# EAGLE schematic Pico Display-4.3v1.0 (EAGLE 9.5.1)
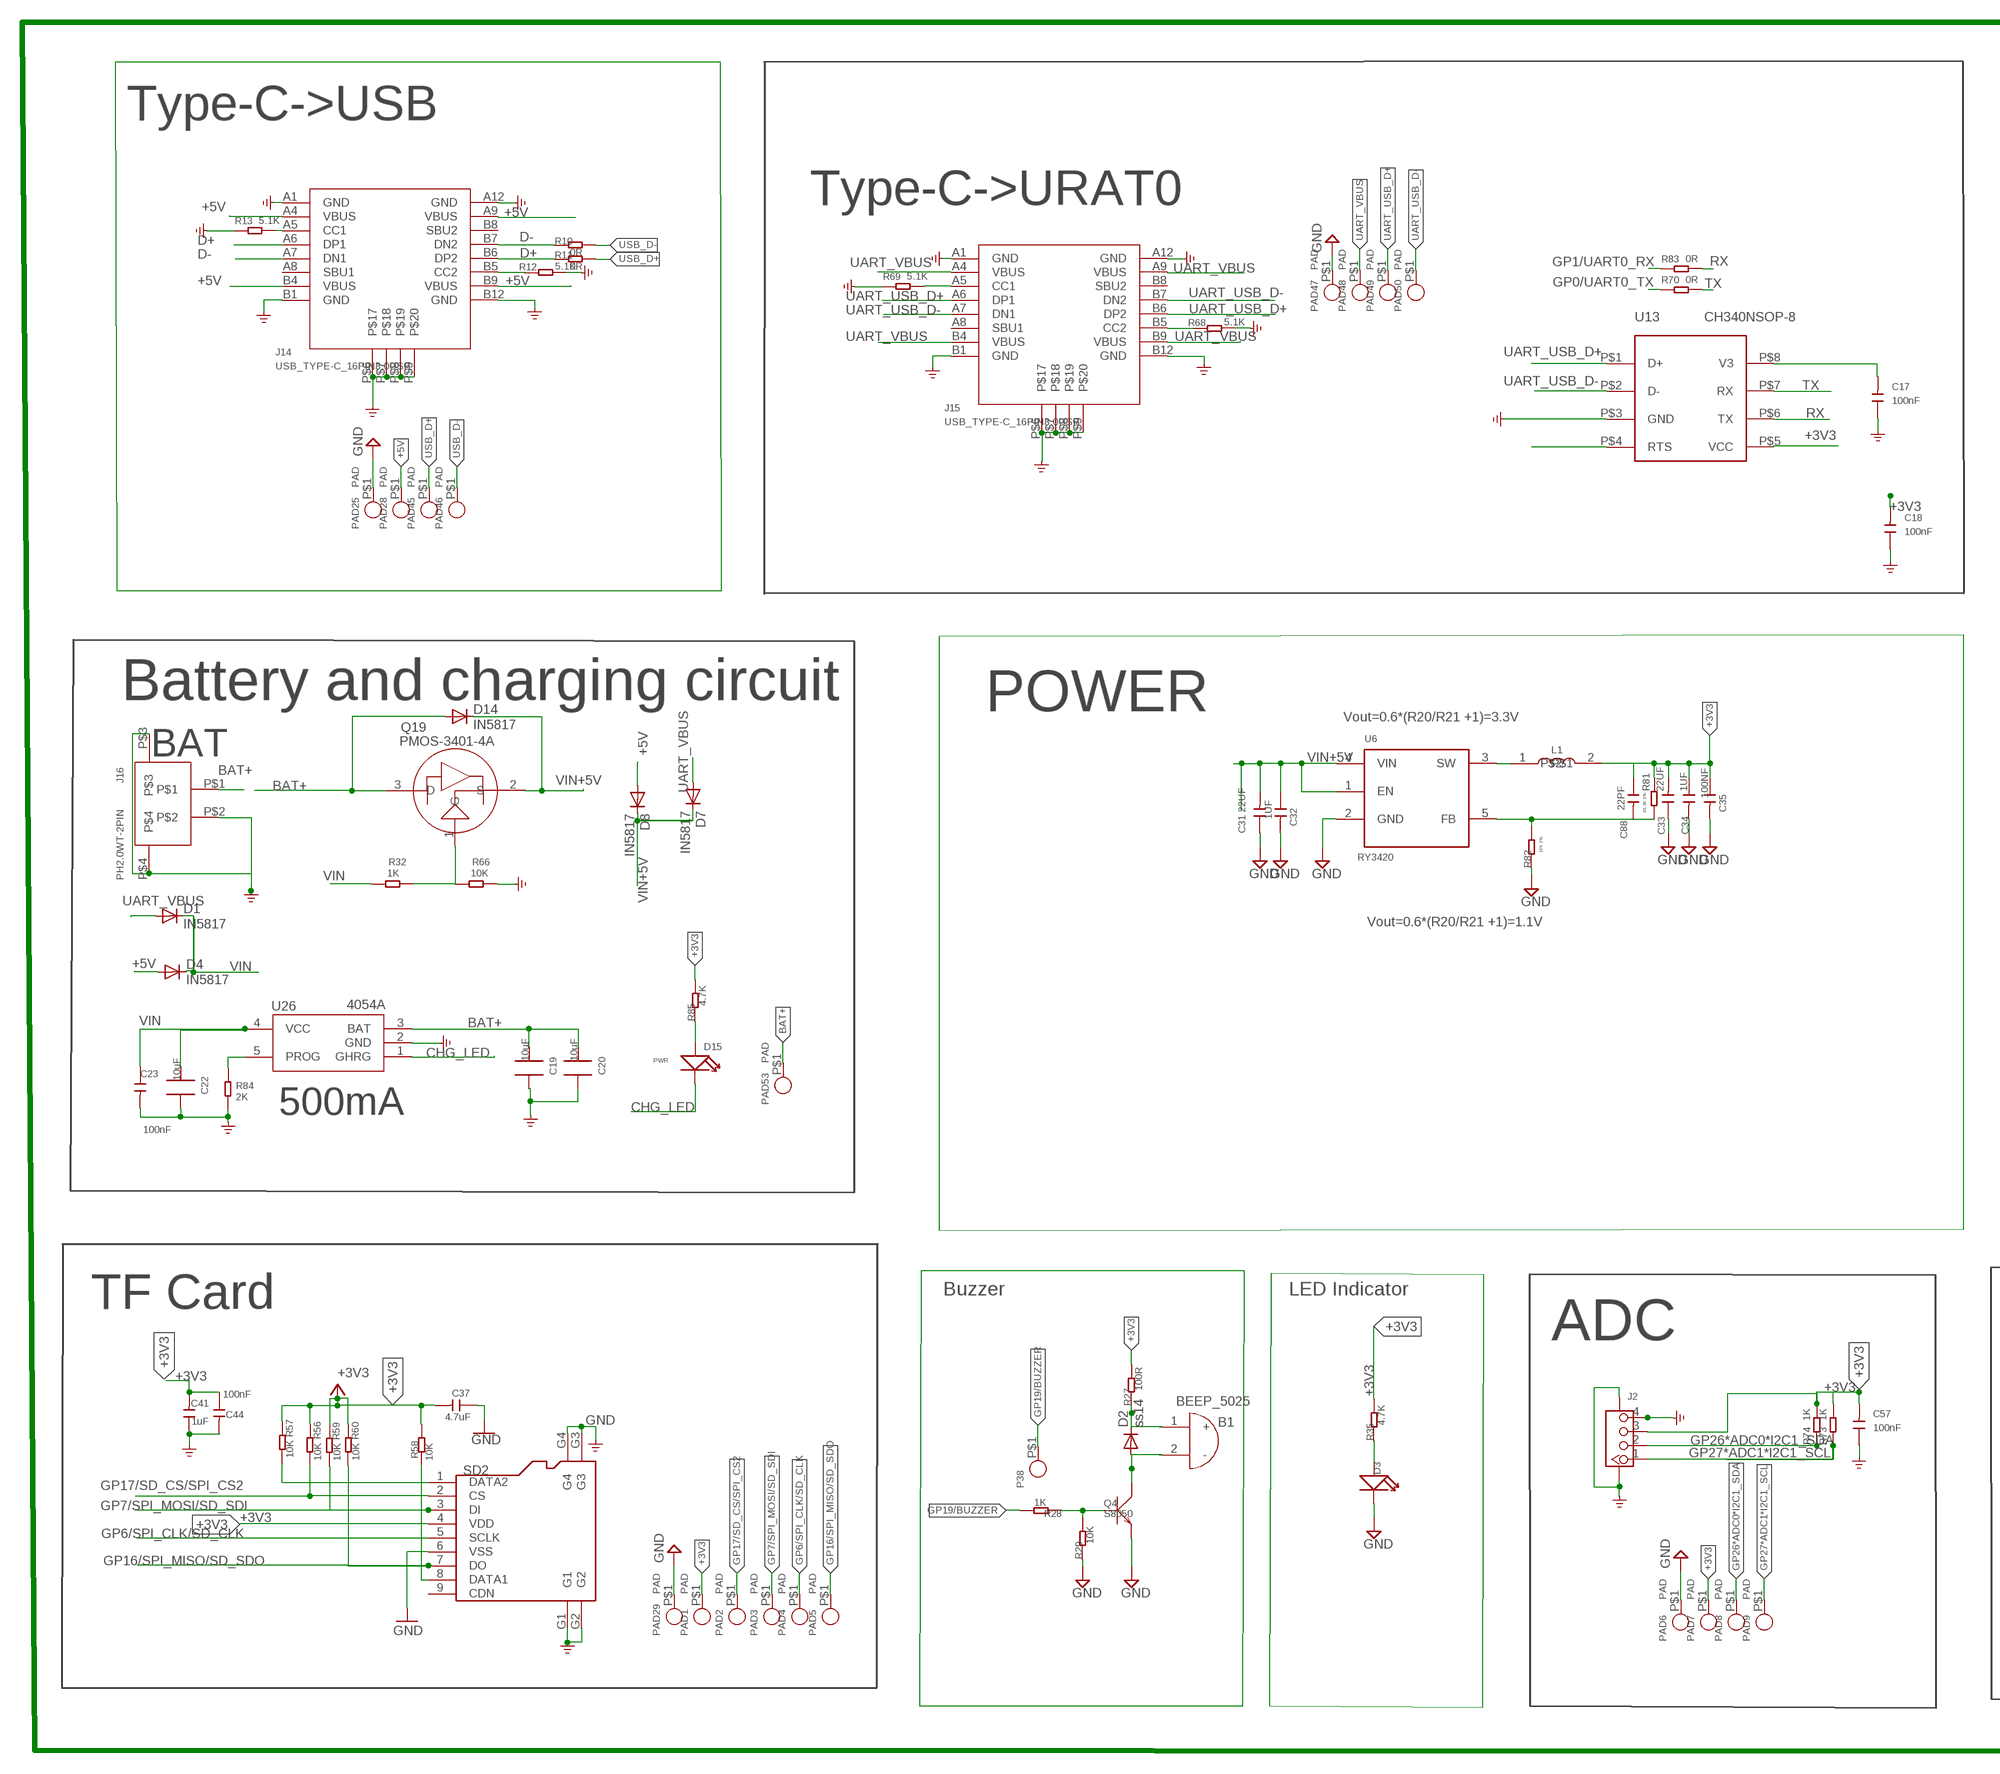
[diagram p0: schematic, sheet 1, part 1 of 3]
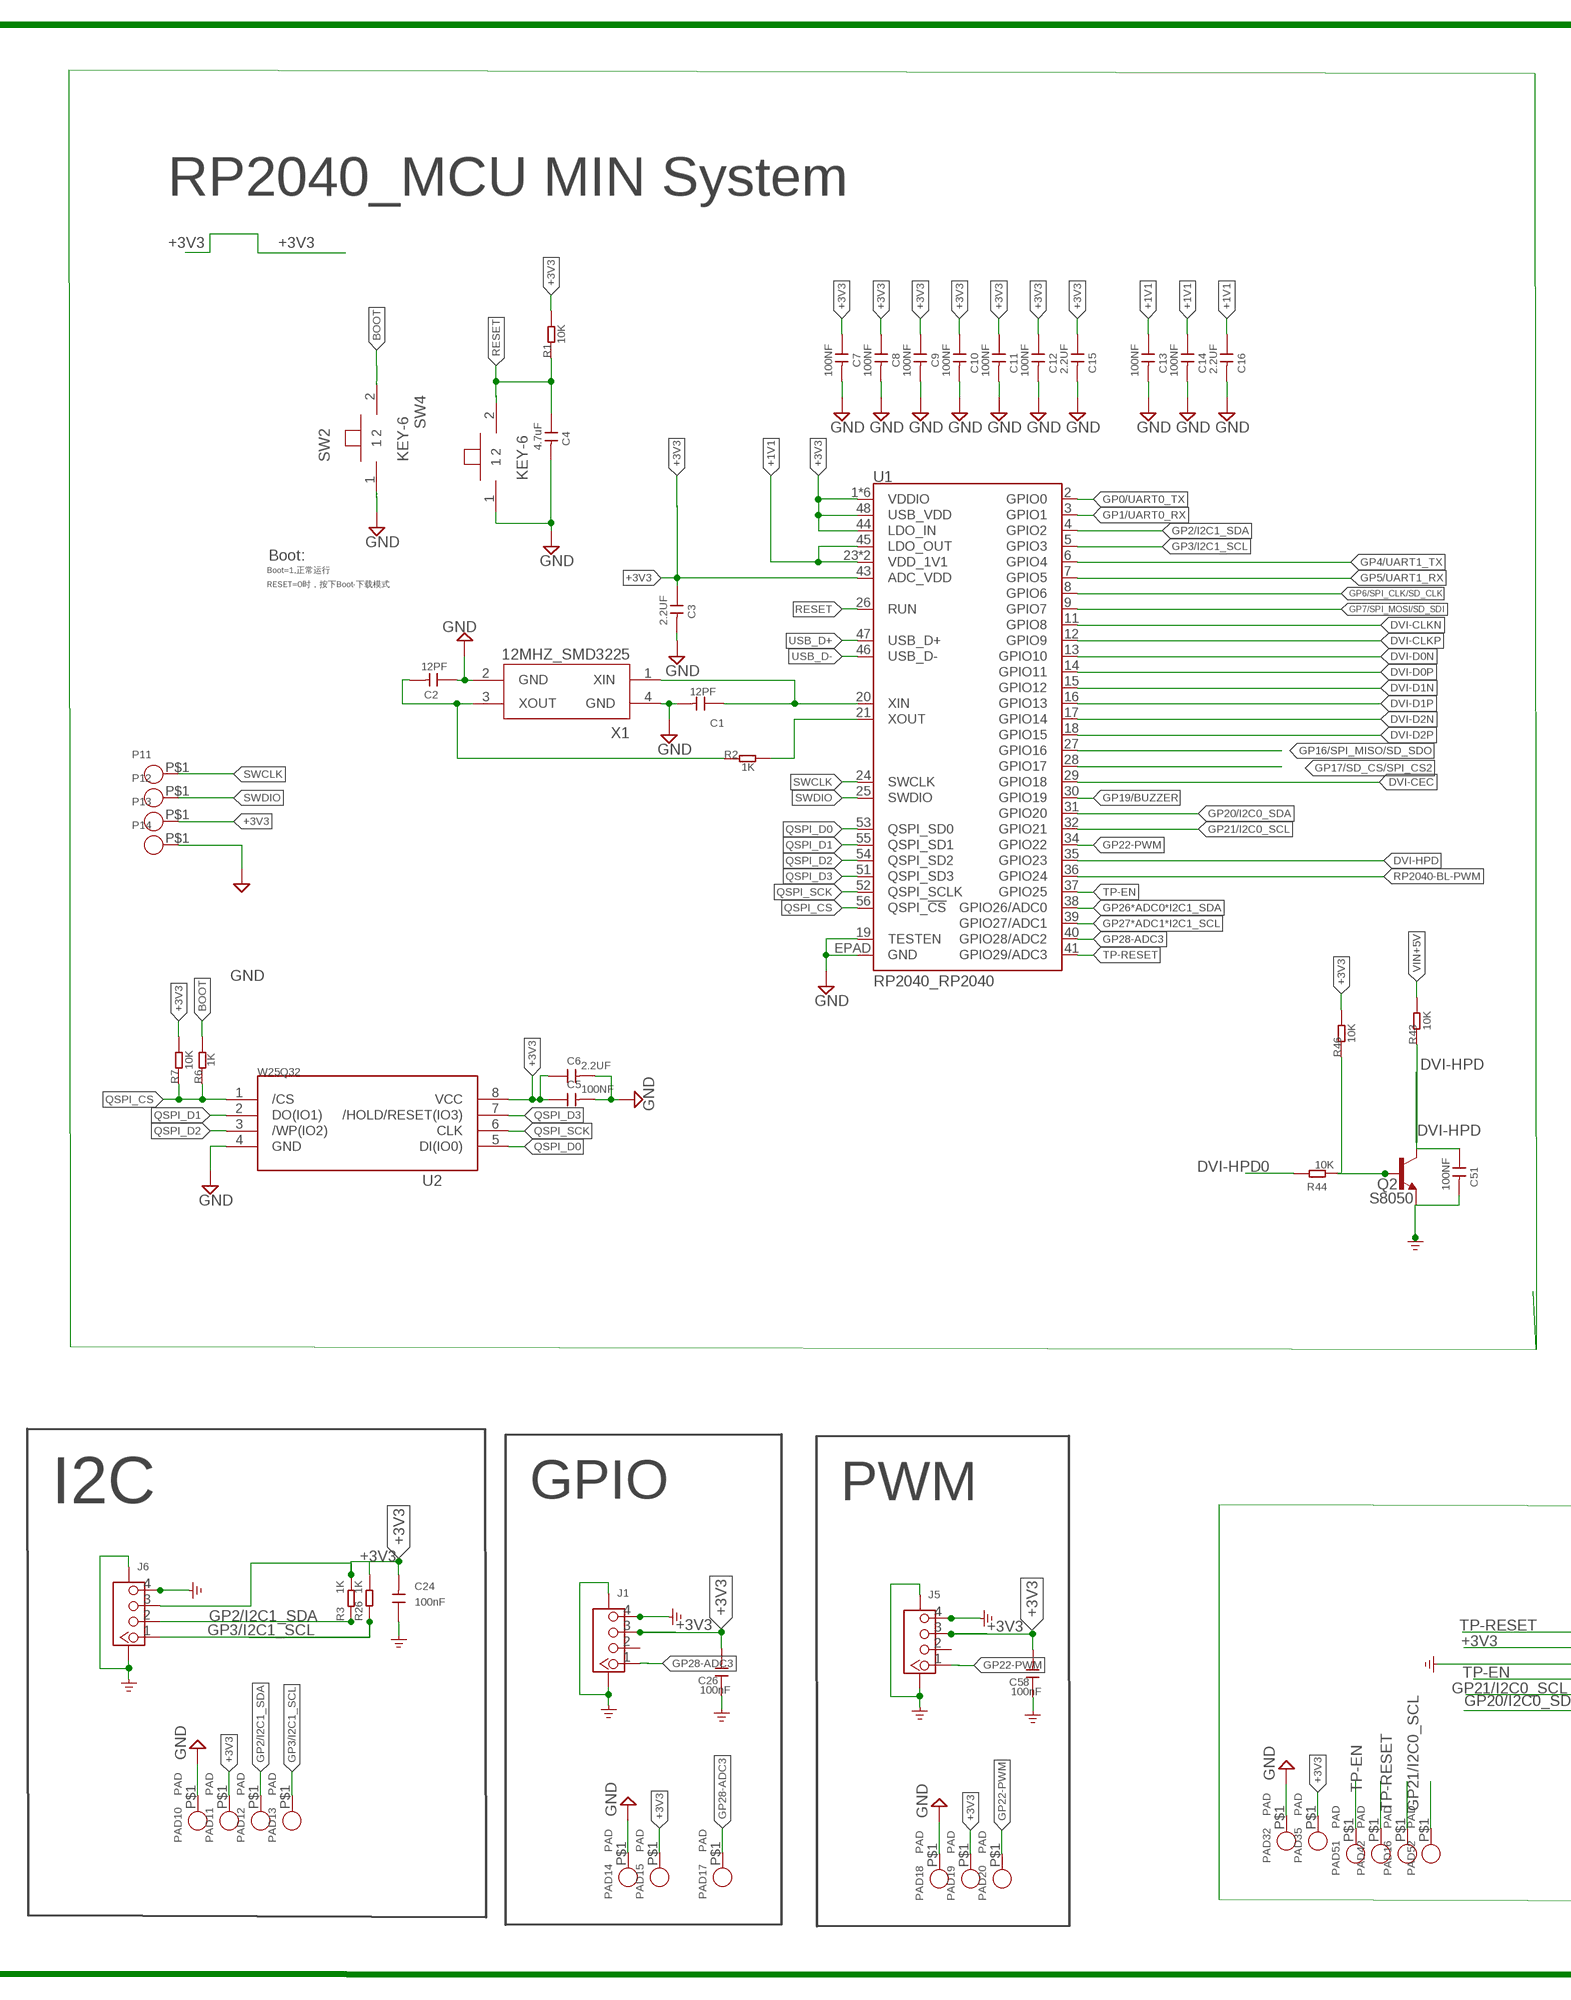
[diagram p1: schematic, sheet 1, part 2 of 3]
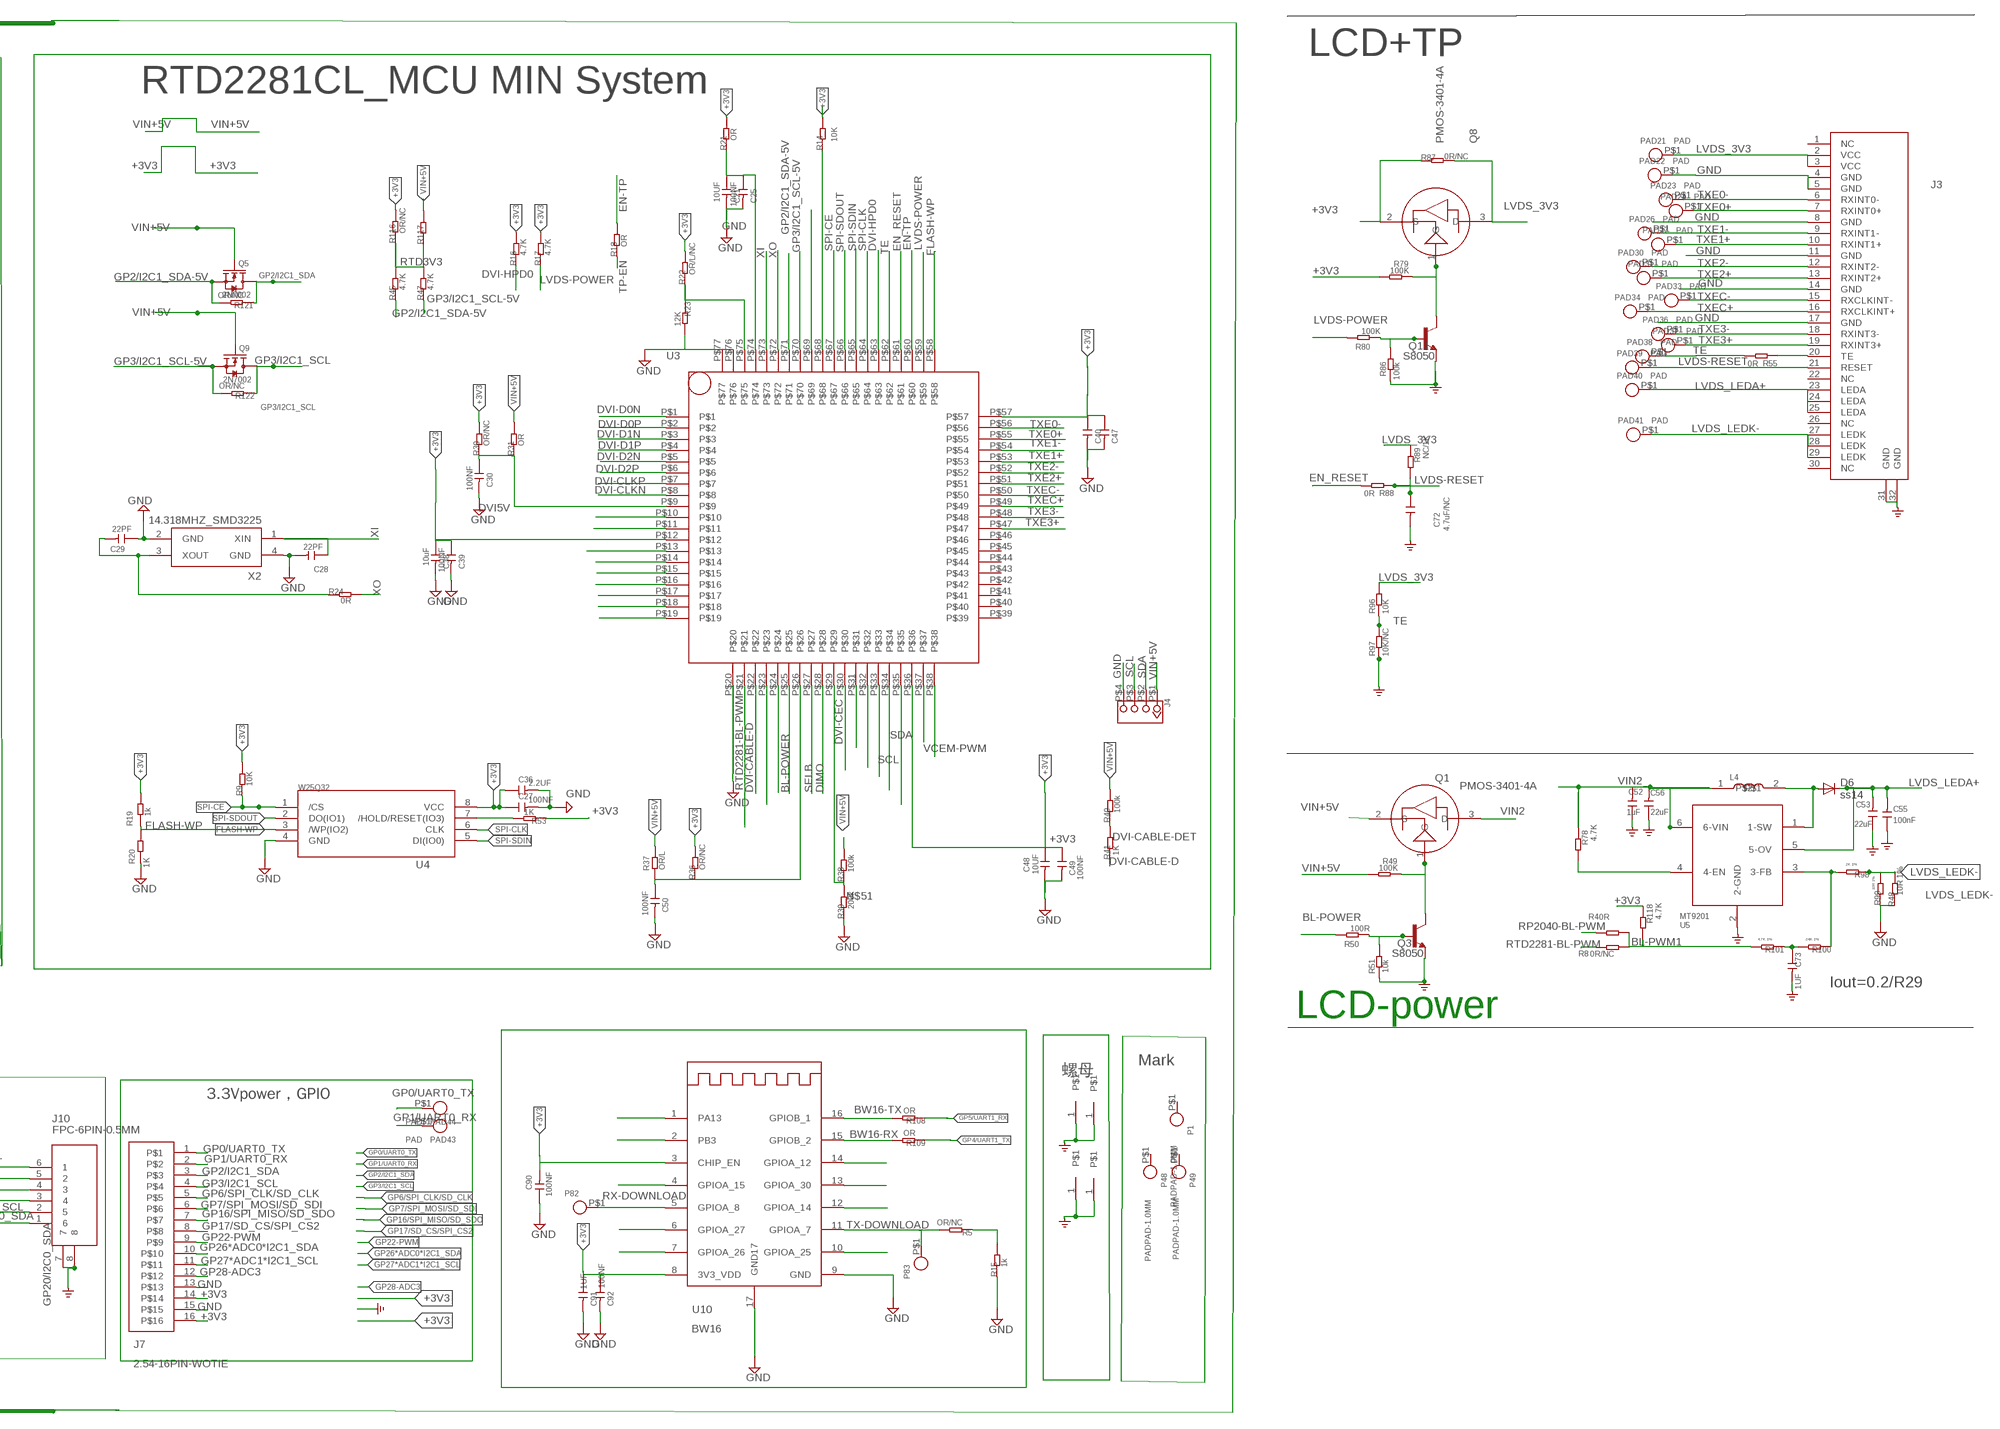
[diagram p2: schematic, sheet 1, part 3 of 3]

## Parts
B1  BEEP_5025  [BEEP_5025]
C1  12PF  A_XBJ_C0603  [A_XBJ_0603]
C2  12PF  A_XBJ_C0603  [A_XBJ_0603]
C3  2.2UF  A_XBJ_C0603  [A_XBJ_0603]
C4  4.7uF  A_XBJ_C0603  [A_XBJ_0603]
C5  100NF  A_XBJ_C0603  [A_XBJ_0603]
C6  2.2UF  A_XBJ_C0603  [A_XBJ_0603]
C7  100NF  A_XBJ_C0603  [A_XBJ_0603]
C8  100NF  A_XBJ_C0603  [A_XBJ_0603]
C9  100NF  A_XBJ_C0603  [A_XBJ_0603]
C10  100NF  A_XBJ_C0603  [A_XBJ_0603]
C11  100NF  A_XBJ_C0603  [A_XBJ_0603]
C12  100NF  A_XBJ_C0603  [A_XBJ_0603]
C13  100NF  A_XBJ_C0603  [A_XBJ_0603]
C14  100NF  A_XBJ_C0603  [A_XBJ_0603]
C15  2.2UF  A_XBJ_C0603  [A_XBJ_0603]
C16  2.2UF  A_XBJ_C0603  [A_XBJ_0603]
C17  100nF  C0603  [0603]
C18  100nF  C0603  [0603]
C19  10uF  C0805_S  [0805_S]
C20  10uF  C0805_S  [0805_S]
C21  10UF  A_XBJ_C0603  [A_XBJ_0603]
C22  10uF  C0805_S  [0805_S]
C23  100nF  C-0603  [C0603]
C24  100nF  C0603  [0603]
C25  100NF  A_XBJ_C0603  [A_XBJ_0603]
C26  100nF  C0603  [0603]
C27  100NF  A_XBJ_C0603  [A_XBJ_0603]
C28  22PF  A_XBJ_C0603  [A_XBJ_0603]
C29  22PF  A_XBJ_C0603  [A_XBJ_0603]
C30  100NF  A_XBJ_C0603  [A_XBJ_0603]
C31  22UF  A_XBJ_C0805  [A_XBJ_0805]
C32  1UF  A_XBJ_C0603  [A_XBJ_0603]
C33  22UF  A_XBJ_C0805  [A_XBJ_0805]
C34  1UF  A_XBJ_C0603  [A_XBJ_0603]
C35  100NF  A_XBJ_C0603  [A_XBJ_0603]
C36  2.2UF  A_XBJ_C0603  [A_XBJ_0603]
C37  4.7uF  DISCRETE_C-0603  [DISCRETE_C0603]
C38  10uF  A_XBJ_C0603  [A_XBJ_0603]
C39  100NF  A_XBJ_C0603  [A_XBJ_0603]
C40  10UF  A_XBJ_C0603  [A_XBJ_0603]
C41  1uF  DISCRETE_C-0603  [DISCRETE_C0603]
C44  100nF  C-0603  [C0603]
C47  100NF  A_XBJ_C0603  [A_XBJ_0603]
C48  10UF  A_XBJ_C0603  [A_XBJ_0603]
C49  100NF  A_XBJ_C0603  [A_XBJ_0603]
C50  100NF  A_XBJ_C0603  [A_XBJ_0603]
C51  100NF  A_XBJ_C0603  [A_XBJ_0603]
C52  1uF  C0603  [0603]
C53  22uF  C0805  [0805]
C55  100nF  C0603  [0603]
C56  22uF  C0805  [0805]
C57  100nF  C0603  [0603]
C58  100nF  C0603  [0603]
C72  4.7uF/NC  C0603  [0603]
C73  1UF  A_XBJ_C0603  [A_XBJ_0603]
C88  22PF  A_XBJ_C0603  [A_XBJ_0603]
C90  100NF  A_XBJ_C0603  [A_XBJ_0603]
C91  1UF  A_XBJ_C0603  [A_XBJ_0603]
C92  100NF  A_XBJ_C0603  [A_XBJ_0603]
D1  IN5817  DIODE-DO-214AC  [DO-214AC]
D2  ss14  DIODE-DO-214AC  [DO-214AC]
D3  DISCRETE_007-LED0603  [DISCRETE_D0603]
D4  IN5817  DIODE-DO-214AC  [DO-214AC]
D6  ss14  DIODE-DO-214AC  [DO-214AC]
D7  IN5817  DIODE-DO-214AC  [DO-214AC]
D8  IN5817  DIODE-DO-214AC  [DO-214AC]
D14  IN5817  DIODE-DO-214AC  [DO-214AC]
D15  DISCRETE_007-LED0603  [DISCRETE_D0603]
J1  CONNECTOR_TWIG-4P-2.0-SMD-FEMALE-REINFORCE90D  [CONNECTOR_4P-SMD-2.0-90D]
J2  CONNECTOR_TWIG-4P-2.0-SMD-FEMALE-REINFORCE90D  [CONNECTOR_4P-SMD-2.0-90D]
J3  FPC-0.5-30P-LVDS  [FPC-30P-0.5]
J4  CON_4PIN_DIP_P2.54  [CON_4PIN_DIP_P2.54]
J5  CONNECTOR_TWIG-4P-2.0-SMD-FEMALE-REINFORCE90D  [CONNECTOR_4P-SMD-2.0-90D]
J6  CONNECTOR_TWIG-4P-2.0-SMD-FEMALE-REINFORCE90D  [CONNECTOR_4P-SMD-2.0-90D]
J7  2.54-16PIN-WOTIE  [2.54-16P-WOTIE]
J10  FPC-6PIN-0.5MM  [FPC-6PIN-0.5MM]
J14  USB_TYPE-C_16PIN3.0USB  [KEVIN_3.0TYPEC-SMD]
J15  USB_TYPE-C_16PIN3.0USB  [KEVIN_3.0TYPEC-SMD]
J16  PH2.0WT-2PIN  [PH2.0WT-2PIN]
L1  L-0530  [CD54_CD54]
L4  L-0530  [CD54_CD54]
P1  PADPAD-1.0MM  [PAD-1.0MM]
P11  CROWPI_POW_PADPAD-1.0MM  [CROWPI_POW_PAD-1.0MM]
P12  CROWPI_POW_PADPAD-1.0MM  [CROWPI_POW_PAD-1.0MM]
P13  CROWPI_POW_PADPAD-1.0MM  [CROWPI_POW_PAD-1.0MM]
P14  CROWPI_POW_PADPAD-1.0MM  [CROWPI_POW_PAD-1.0MM]
P38  CROWPI_POW_PADPAD-1.0MM  [CROWPI_POW_PAD-1.0MM]
P48  PADPAD-1.0MM  [PAD-1.0MM]
P49  PADPAD-1.0MM  [PAD-1.0MM]
P82  CROWPI_POW_PADPAD-1.0MM  [CROWPI_POW_PAD-1.0MM]
P83  CROWPI_POW_PADPAD-1.0MM  [CROWPI_POW_PAD-1.0MM]
PAD1  PAD  [PAD-1.5MM]
PAD2  PAD  [PAD-1.5MM]
PAD3  PAD  [PAD-1.5MM]
PAD4  PAD  [PAD-1.5MM]
PAD5  PAD  [PAD-1.5MM]
PAD6  PAD  [PAD-1.5MM]
PAD7  PAD  [PAD-1.5MM]
PAD8  PAD  [PAD-1.5MM]
PAD9  PAD  [PAD-1.5MM]
PAD10  PAD  [PAD-1.5MM]
PAD11  PAD  [PAD-1.5MM]
PAD12  PAD  [PAD-1.5MM]
PAD13  PAD  [PAD-1.5MM]
PAD14  PAD  [PAD-1.5MM]
PAD15  PAD  [PAD-1.5MM]
PAD16  PAD  [PAD-1.5MM]
PAD17  PAD  [PAD-1.5MM]
PAD18  PAD  [PAD-1.5MM]
PAD19  PAD  [PAD-1.5MM]
PAD20  PAD  [PAD-1.5MM]
PAD21  PAD  [PAD-1.5MM]
PAD22  PAD  [PAD-1.5MM]
PAD23  PAD  [PAD-1.5MM]
PAD24  PAD  [PAD-1.5MM]
PAD25  PAD  [PAD-1.5MM]
PAD26  PAD  [PAD-1.5MM]
PAD27  PAD  [PAD-1.5MM]
PAD28  PAD  [PAD-1.5MM]
PAD29  PAD  [PAD-1.5MM]
PAD30  PAD  [PAD-1.5MM]
PAD31  PAD  [PAD-1.5MM]
PAD32  PAD  [PAD-1.5MM]
PAD33  PAD  [PAD-1.5MM]
PAD34  PAD  [PAD-1.5MM]
PAD35  PAD  [PAD-1.5MM]
PAD36  PAD  [PAD-1.5MM]
PAD37  PAD  [PAD-1.5MM]
PAD38  PAD  [PAD-1.5MM]
PAD39  PAD  [PAD-1.5MM]
PAD40  PAD  [PAD-1.5MM]
PAD41  PAD  [PAD-1.5MM]
PAD42  PAD  [PAD-1.5MM]
PAD43  PAD  [PAD-1.5MM]
PAD44  PAD  [PAD-1.5MM]
PAD45  PAD  [PAD-1.5MM]
PAD46  PAD  [PAD-1.5MM]
PAD47  PAD  [PAD-1.5MM]
PAD48  PAD  [PAD-1.5MM]
PAD49  PAD  [PAD-1.5MM]
PAD50  PAD  [PAD-1.5MM]
PAD51  PAD  [PAD-1.5MM]
PAD52  PAD  [PAD-1.5MM]
PAD53  PAD  [PAD-1.5MM]
Q1  PMOS-3401-4A  P-MOS-SOT23  [SOT-23]
Q2  S8050  SPARKFUN_TRANSISTOR_NPNSOT23  [SPARKFUN_SOT23]
Q3  S8050  SPARKFUN_TRANSISTOR_NPNSOT23  [SPARKFUN_SOT23]
Q4  S8050  DISCRETE_TRANSISTOR-NPN-SOT23  [DISCRETE_SOT23$1]
Q5  2N7002  MOSFET-N'SOT23'  [SOT23]
Q8  PMOS-3401-4A  P-MOS-SOT23  [SOT-23]
Q9  2N7002  MOSFET-N'SOT23'  [SOT23]
Q11  S8050  SPARKFUN_TRANSISTOR_NPNSOT23  [SPARKFUN_SOT23]
Q19  PMOS-3401-4A  P-MOS-SOT23  [SOT-23]
R1  10K  DISCRETE_R-0603  [DISCRETE_R0603]
R2  1K  DISCRETE_R-0603  [DISCRETE_R0603]
R3  1K  DISCRETE_R-0603  [DISCRETE_R0603]
R4  0R  DISCRETE_R-0603  [DISCRETE_R0603]
R5  OR/NC  DISCRETE_R-0603  [DISCRETE_R0603]
R6  1K  DISCRETE_R-0603  [DISCRETE_R0603]
R7  10K  DISCRETE_R-0603  [DISCRETE_R0603]
R8  0R/NC  DISCRETE_R-0603  [DISCRETE_R0603]
R9  10K  DISCRETE_R-0603  [DISCRETE_R0603]
R10  0R  DISCRETE_R-0603  [DISCRETE_R0603]
R11  0R  DISCRETE_R-0603  [DISCRETE_R0603]
R12  5.1K  DISCRETE_R-0603  [DISCRETE_R0603]
R13  5.1K  DISCRETE_R-0603  [DISCRETE_R0603]
R14  10K  DISCRETE_R-0603  [DISCRETE_R0603]
R15  1k  DISCRETE_R-0603  [DISCRETE_R0603]
R16  4.7K  DISCRETE_R-0603  [DISCRETE_R0603]
R17  4.7K  DISCRETE_R-0603  [DISCRETE_R0603]
R18  OR  DISCRETE_R-0603  [DISCRETE_R0603]
R19  1k  DISCRETE_R-0603  [DISCRETE_R0603]
R20  1K  DISCRETE_R-0603  [DISCRETE_R0603]
R21  OR  DISCRETE_R-0603  [DISCRETE_R0603]
R22  OR/L/NC  DISCRETE_R-0603  [DISCRETE_R0603]
R23  12K  DISCRETE_R-0603  [DISCRETE_R0603]
R24  0R  DISCRETE_R-0603  [DISCRETE_R0603]
R26  1K  DISCRETE_R-0603  [DISCRETE_R0603]
R27  100R  DISCRETE_R-0603  [DISCRETE_R0603]
R28  1K  DISCRETE_R-0603  [DISCRETE_R0603]
R29  10K  DISCRETE_R-0603  [DISCRETE_R0603]
R30  OR/NC  DISCRETE_R-0603  [DISCRETE_R0603]
R31  OR  DISCRETE_R-0603  [DISCRETE_R0603]
R32  1K  DISCRETE_R-0603  [DISCRETE_R0603]
R35  4.7K  DISCRETE_R-0603  [DISCRETE_R0603]
R36  OR/NC  DISCRETE_R-0603  [DISCRETE_R0603]
R37  OR/L  DISCRETE_R-0603  [DISCRETE_R0603]
R38  100k  DISCRETE_R-0603  [DISCRETE_R0603]
R39  200k  DISCRETE_R-0603  [DISCRETE_R0603]
R40  100k  DISCRETE_R-0603  [DISCRETE_R0603]
R41  1K  DISCRETE_R-0603  [DISCRETE_R0603]
R43  10K  DISCRETE_R-0603  [DISCRETE_R0603]
R44  10K  R0603  [R0603]
R45  4.7K  DISCRETE_R-0603  [DISCRETE_R0603]
R46  10K  DISCRETE_R-0603  [DISCRETE_R0603]
R47  4.7K  DISCRETE_R-0603  [DISCRETE_R0603]
R48  10R 1%  DISCRETE_R-0603  [DISCRETE_R0603]
R49  100K  R-0603  [R0603]
R50  100R  R0603  [R0603]
R51  10k  R0603  [R0603]
R53  1K  DISCRETE_R-0603  [DISCRETE_R0603]
R55  0R  DISCRETE_R-0603  [DISCRETE_R0603]
R56  10K  DISCRETE_R-0603  [DISCRETE_R0603]
R57  10K  DISCRETE_R-0603  [DISCRETE_R0603]
R58  10K  DISCRETE_R-0603  [DISCRETE_R0603]
R59  10K  DISCRETE_R-0603  [DISCRETE_R0603]
R60  10K  DISCRETE_R-0603  [DISCRETE_R0603]
R66  10K  DISCRETE_R-0603  [DISCRETE_R0603]
R68  5.1K  DISCRETE_R-0603  [DISCRETE_R0603]
R69  5.1K  DISCRETE_R-0603  [DISCRETE_R0603]
R70  0R  DISCRETE_R-0603  [DISCRETE_R0603]
R73  1K  DISCRETE_R-0603  [DISCRETE_R0603]
R74  1K  DISCRETE_R-0603  [DISCRETE_R0603]
R78  4.7K  DISCRETE_R-0603  [DISCRETE_R0603]
R79  100K  R-0603  [R0603]
R80  100K  R0603  [R0603]
R81  45.3K 1%  DISCRETE_R-0603  [DISCRETE_R0603]
R82  10K 1%  DISCRETE_R-0603  [DISCRETE_R0603]
R83  0R  DISCRETE_R-0603  [DISCRETE_R0603]
R84  2K  DISCRETE_R-0603  [DISCRETE_R0603]
R85  4.7K  DISCRETE_R-0603  [DISCRETE_R0603]
R86  100k  R0603  [R0603]
R87  0R/NC  DISCRETE_R-0603  [DISCRETE_R0603]
R88  0R  DISCRETE_R-0603  [DISCRETE_R0603]
R89  NC/1K  DISCRETE_R-0603  [DISCRETE_R0603]
R96  10K  DISCRETE_R-0603  [DISCRETE_R0603]
R97  10K/NC  DISCRETE_R-0603  [DISCRETE_R0603]
R98  2K 1%  DISCRETE_R-0603  [DISCRETE_R0603]
R99  10R 1%  DISCRETE_R-0603  [DISCRETE_R0603]
R100  24K 1%  DISCRETE_R-0603  [DISCRETE_R0603]
R101  4.7K 1%  DISCRETE_R-0603  [DISCRETE_R0603]
R108  OR  DISCRETE_R-0603  [DISCRETE_R0603]
R109  OR  DISCRETE_R-0603  [DISCRETE_R0603]
R116  OR/NC  DISCRETE_R-0603  [DISCRETE_R0603]
R117  0R  DISCRETE_R-0603  [DISCRETE_R0603]
R118  4.7K  DISCRETE_R-0603  [DISCRETE_R0603]
R121  OR/NC  DISCRETE_R-0603  [DISCRETE_R0603]
R122  OR/NC  DISCRETE_R-0603  [DISCRETE_R0603]
SD2  HOLDER-MICROSD-9P  [9P-SMD-W/-RING]
SW2  KEY-6  [KEY-6]
SW4  KEY-6  [KEY-6]
T1  3M-5  [3M-5]
T2  3M-5  [3M-5]
T3  3M-5  [3M-5]
T4  3M-5  [3M-5]
U1  RP2040_RP2040  [RP2040_QFN-56]
U2  SELF_W25Q128JV  [SELF_SOIC-8-208MIL]
U3  RTD2281CL  [RTD2281CL-MQFN-76]
U4  SELF_W25Q128JV  [SELF_SOIC-8-208MIL]
U5  MT9201  [SOT23-6]
U6  RY3420  CROWBOT_-V1.0-20220525_A_XBJ_HM3420B  [CROWBOT_-V1.0-20220525_A_XBJ_SOT23-5]
U10  BW16  [BW16]
U13  CH340NSOP-8  [SOP8]
U26  4054A  [SOP23-5]
X1  12MHZ_SMD3225  A_XBJ_XTAL  [A_XBJ_SMD3225]
X2  14.318MHZ_SMD3225  A_XBJ_XTAL  [A_XBJ_SMD3225]

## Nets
+1V1: C13.1 C14.1 C16.1 U1.23(VDD_1V1) U1.45(LDO_OUT) U1.50(VDD_1V1)
+3V3: C3.1 C5.1 C6.1 C7.1 C8.1 C9.1 C10.1 C11.1 C12.1 C15.1 C18.2 C24.2 C26.2 C27.1 C33.2 C34.1 C35.1 C36.1 C37.2 C38.1 C39.1 C40.1 C41.2 C44.1 C47.1 C48.1 C49.1 C57.2 C58.2 C88.1 C90.2 C91.1 C92.1 J1.3 J2.3 J5.3 J6.3 J7.14 J7.16 J10.5 L1.2 P13.P$1 PAD1.P$1 PAD7.P$1 PAD11.P$1 PAD15.P$1 PAD19.P$1 PAD35.P$1 Q8.2(S) R1.2 R3.2 R7.2 R9.2 R14.2 R16.2 R17.2 R19.2 R21.2 R22.2 R26.2 R27.2 R30.2 R35.2 R36.2 R46.2 R53.1 R56.1 R57.1 R58.1 R59.1 R60.1 R73.2 R74.2 R79.1 R81.1 R85.2 R87.1 R116.2 R118.2 SD2.4(VDD) U1.1(VDDIO) U1.10(VDDIO) U1.22(VDDIO) U1.33(VDDIO) U1.42(VDDIO) U1.43(ADC_VDD) U1.44(LDO_IN) U1.48(USB_VDD) U1.49(VDDIO) U2.8(VCC) U3.P$12 U3.P$36 U3.P$57 U4.8(VCC) U10.3(CHIP_EN) U10.8(3V3_VDD) U13.P$5(VCC)
+5V [PWR]: D4.A D8.A J14.A4(VBUS) J14.A9(VBUS) J14.B4(VBUS) J14.B9(VBUS) PAD28.P$1
BAT+: C19.2 C20.2 D14.A J16.P$1 PAD53.P$1 Q19.3(D) U26.3(BAT)
BL-POWER: R50.2 U3.P$25
BL-PWM1: R4.1 R8.1 R101.2 R118.1
BOOT: R6.2 SW2.2
BW16-RX: R109.2 U10.15(GPIOB_2)
BW16-TX: R108.2 U10.16(GPIOB_1)
CHG_LED: D15.- U26.1(GHRG)
D+ [USB]: J14.A6(DP1) J14.B6(DP2) R11.1
D- [USB]: J14.A7(DN1) J14.B7(DN2) R10.1
DIMO: U3.P$28
DVI5V: C30.1 R30.1 R31.1 U3.P$9
DVI-CABLE-D: R41.1 U3.P$22
DVI-CABLE-DET: R40.1 R41.2
DVI-CEC: U1.29(GPIO18) U3.P$30
DVI-CLKN: U1.11(GPIO8) U3.P$8
DVI-CLKP: U1.12(GPIO9) U3.P$7
DVI-D0N: U1.13(GPIO10) U3.P$1
DVI-D0P: U1.14(GPIO11) U3.P$2
DVI-D1N: U1.15(GPIO12) U3.P$3
DVI-D1P: U1.16(GPIO13) U3.P$4
DVI-D2N: U1.17(GPIO14) U3.P$5
DVI-D2P: U1.18(GPIO15) U3.P$6
DVI-HPD: C51.1 Q2.3(C) R43.1 U1.35(GPIO23)
DVI-HPD0: R16.1 R44.2 U3.P$63
EN-TP: R18.2 U3.P$60
EN_RESET: R88.2 U3.P$61
FLASH-WP: R19.1 R20.2 U3.P$58 U4.3(/WP(IO2))
GND [GND]: C1.2 C2.1 C3.2 C4.2 C5.2 C6.2 C7.2 C8.2 C9.2 C10.2 C11.2 C12.2 C13.2 C14.2 C15.2 C16.2 C17.1 C18.1 C19.1 C20.1 C21.2 C22.1 C23.2 C24.1 C25.2 C26.1 C27.2 C28.2 C29.1 C30.2 C31.1 C32.2 C33.1 C34.2 C35.2 C36.2 C37.1 C38.2 C39.2 C40.2 C41.1 C44.2 C47.2 C48.2 C49.2 C50.2 C51.2 C52.1 C53.1 C55.1 C56.1 C57.1 C58.1 C72.2 C73.2 C90.1 C91.2 C92.2 D3.- J1.4 J1.SS1 J1.SS2 J2.4 J2.SS1 J2.SS2 J3.4(GND) J3.5(GND) J3.8(GND) J3.11(GND) J3.14(GND) J3.17(GND) J3.31(GND) J3.32(GND) J4.P$4 J5.4 J5.SS1 J5.SS2 J6.4 J6.SS1 J6.SS2 J7.13 J7.15 J10.4 J10.7 J10.8 J14.A1(GND) J14.A12(GND) J14.B1(GND) J14.B12(GND) J14.P$6 J14.P$7 J14.P$8 J14.P$9 J15.A1(GND) J15.A12(GND) J15.B1(GND) J15.B12(GND) J15.P$6 J15.P$7 J15.P$8 J15.P$9 J16.P$2 J16.P$3 J16.P$4 P14.P$1 PAD6.P$1 PAD10.P$1 PAD14.P$1 PAD18.P$1 PAD22.P$1 PAD25.P$1 PAD29.P$1 PAD32.P$1 PAD47.P$1 Q2.2(E) Q3.2(E) Q4.2(E) Q11.2(E) R12.2 R13.1 R15.1 R20.1 R23.2 R29.1 R39.1 R48.2 R51.1 R66.1 R68.2 R69.1 R82.1 R84.2 R86.1 R97.1 R99.1 SD2.6(VSS) SD2.G1 SD2.G2 SD2.G3 SD2.G4 SW2.1 SW4.1 T1.1 T2.1 T3.1 T4.1 U1.19(TESTEN) U1.EPAD(GND) U2.4(GND) U3.P$20 U3.P$76 U3.P$77 U4.4(GND) U5.2(2-GND) U6.2(GND) U10.9(GND) U10.17(GND17) U13.P$3(GND) U26.2(GND) X1.2(GND) X1.4(GND) X2.2(GND) X2.4(GND)
GP0/UART0_TX: J7.1 PAD44.P$1 R70.1 U1.2(GPIO0)
GP1/UART0_RX: J7.2 PAD43.P$1 R83.1 U1.3(GPIO1)
GP2/I2C1_SDA: J6.2 J7.3 PAD12.P$1 Q5.3(D) R3.1 R121.1 U1.4(GPIO2)
GP2/I2C1_SDA-5V: Q5.2(S) R45.1 R121.2 U3.P$71
GP3/I2C1_SCL: J6.1 J7.4 PAD13.P$1 Q9.3(D) R26.1 R122.1 U1.5(GPIO3)
GP3/I2C1_SCL-5V: Q9.2(S) R47.1 R122.2 U3.P$70
GP4/UART1_TX: R109.1 U1.6(GPIO4)
GP5/UART1_RX: R108.1 U1.7(GPIO5)
GP6/SPI_CLK/SD_CLK: J7.5 PAD4.P$1 SD2.5(SCLK) U1.8(GPIO6)
GP7/SPI_MOSI/SD_SDI: J7.6 PAD3.P$1 R59.2 SD2.3(DI) U1.9(GPIO7)
GP16/SPI_MISO/SD_SDO: J7.7 PAD5.P$1 R60.2 SD2.7(DO) U1.27(GPIO16)
GP17/SD_CS/SPI_CS2: J7.8 PAD2.P$1 R56.2 SD2.2(CS) U1.28(GPIO17)
GP19/BUZZER: P38.P$1 R28.2 U1.30(GPIO19)
GP20/I2C0_SDA: J10.1 PAD52.P$1 U1.31(GPIO20)
GP21/I2C0_SCL: J10.2 PAD16.P$1 U1.32(GPIO21)
GP22-PWM: J5.1 J7.9 PAD20.P$1 U1.34(GPIO22)
GP26*ADC0*I2C1_SDA: J2.2 J7.10 PAD8.P$1 R74.1 U1.38(GPIO26/ADC0)
GP27*ADC1*I2C1_SCL: J2.1 J7.11 PAD9.P$1 R73.1 U1.39(GPIO27/ADC1)
GP28-ADC3: J1.1 J7.12 PAD17.P$1 U1.40(GPIO28/ADC2)
LVDS-POWER: R17.1 R80.2 U3.P$59
LVDS-RESET: C72.1 J3.21(RESET) PAD39.P$1 R88.1 R89.1
LVDS_3V3: J3.2(VCC) J3.3(VCC) PAD21.P$1 Q8.3(D) R87.2 R89.2 R96.2
LVDS_LEDA+: C53.2 C55.2 D6.C J3.23(LEDA) J3.24(LEDA) J3.25(LEDA) PAD40.P$1 U5.5(5-OV)
LVDS_LEDK-: J3.27(LEDK) J3.28(LEDK) J3.29(LEDK) PAD41.P$1 R48.1 R98.1 R99.2
N$1: C2.2 R2.1 X1.3(XOUT)
N$2: R2.2 U1.21(XOUT)
N$3: C1.1 U1.20(XIN) X1.1(XIN)
N$5: J15.B5(CC2) R68.1
N$8: J3.20(TE) R55.1
N$9: R84.1 U26.5(PROG)
N$10: L1.1 U6.3(SW)
N$11: U3.P$10
N$14: R53.2 U4.7(/HOLD/RESET(IO3))
N$15: D15.+ R85.1
N$16: J15.A5(CC1) R69.2
N$20: U3.P$38
N$23: Q4.1(B) R28.1 R29.2
N$27: Q19.1(G) R32.1 R66.2
N$28: J14.B5(CC2) R12.1
N$29: B1.2(-) D2.A Q4.3(C)
N$30: B1.1(+) D2.C R27.1
N$31: R98.2 R100.1 U5.3(3-FB)
N$32: J14.A5(CC1) R13.2
N$33: U3.P$11
N$35: D3.+ R35.1
N$36: R57.2 SD2.1(DATA2)
N$39: U3.P$13
N$40: U3.P$14
N$41: U3.P$15
N$42: U3.P$16
N$43: C88.2 R81.2 R82.2 U6.5(FB)
N$44: U3.P$17
N$45: U3.P$18
N$47: U3.P$19
N$49: C73.1 R100.2 R101.1
N$50: C17.2 U13.P$8(V3)
N$51: R38.1 R39.2 U3.P$29
N$52: U3.P$23
N$53: U3.P$24
N$56: U13.P$4(RTS)
N$57: R58.2 SD2.8(DATA1)
N$61: U10.14(GPIOA_12)
N$62: U3.P$31
N$64: U3.P$32
N$65: U10.13(GPIOA_30)
N$66: U3.P$35
N$67: C21.1 C25.1 R21.1 U3.P$74
N$69: U10.12(GPIOA_14)
N$70: D6.A L4.2 U5.1(1-SW)
N$71: Q1.1(G) Q3.3(C) R49.2
N$73: Q3.1(B) R50.1 R51.2
N$74: U10.10(GPIOA_25)
N$76: R5.1 R15.2
N$77: U10.7(GPIOA_26)
N$78: U10.6(GPIOA_27)
N$81: U10.4(GPIOA_15)
N$87: U10.2(PB3)
N$88: U10.1(PA13)
N$99: U3.P$69
N$101: C50.1 R36.1 R37.1 U3.P$26
N$102: C29.2 R24.1 X2.3(XOUT)
N$103: R22.1 R23.1 U3.P$75
N$105: R78.1 U5.4(4-EN)
N$121: Q8.1(G) Q11.3(C) R79.2
N$122: Q11.1(B) R80.1 R86.2
QSPI_CS: R6.1 R7.1 U1.56(QSPI_!CS!) U2.1(/CS)
QSPI_D0: U1.53(QSPI_SD0) U2.5(DI(IO0))
QSPI_D1: U1.55(QSPI_SD1) U2.2(DO(IO1))
QSPI_D2: U1.54(QSPI_SD2) U2.3(/WP(IO2))
QSPI_D3: U1.51(QSPI_SD3) U2.7(/HOLD/RESET(IO3))
QSPI_SCK: U1.52(QSPI_SCLK) U2.6(CLK)
RESET: C4.1 R1.1 SW4.2 U1.26(RUN)
RP2040-BL-PWM: R4.2 U1.36(GPIO24)
RTD3V1: R14.1 U3.P$68
RTD3V3: R45.2 R47.2 R116.1 R117.1
RTD2281-BL-PWM: R8.2 U3.P$21
RX: R83.2 U13.P$6(TX)
RX-DOWNLOAD: P82.P$1 U10.5(GPIOA_8)
SCL: J4.P$3 U3.P$33
SDA: J4.P$2 U3.P$34
SELB: U3.P$27
SPI-CE: R9.1 U3.P$67 U4.1(/CS)
SPI-CLK: U3.P$64 U4.6(CLK)
SPI-SDIN: U3.P$65 U4.5(DI(IO0))
SPI-SDOUT: U3.P$66 U4.2(DO(IO1))
SWCLK: P11.P$1 U1.24(SWCLK)
SWDIO: P12.P$1 U1.25(SWDIO)
TE: PAD38.P$1 R55.2 R96.1 R97.2 U3.P$62
TMDS3V1: Q2.1(B) R44.1 R46.1
TP-EN: J10.3 PAD51.P$1 R18.1 U1.37(GPIO25)
TP-RESET: J10.6 PAD42.P$1 U1.41(GPIO29/ADC3)
TX: R70.2 U13.P$7(RX)
TX-DOWNLOAD: P83.P$1 R5.2 U10.11(GPIOA_7)
TXE0+: J3.7(RXINT0+) PAD24.P$1 U3.P$55
TXE0-: J3.6(RXINT0-) PAD23.P$1 U3.P$56
TXE1+: J3.10(RXINT1+) PAD27.P$1 U3.P$53
TXE1-: J3.9(RXINT1-) PAD26.P$1 U3.P$54
TXE2+: J3.13(RXINT2+) PAD31.P$1 U3.P$51
TXE2-: J3.12(RXINT2-) PAD30.P$1 U3.P$52
TXE3+: J3.19(RXINT3+) PAD37.P$1 U3.P$47
TXE3-: J3.18(RXINT3-) PAD36.P$1 U3.P$48
TXEC+: J3.16(RXCLKINT+) PAD34.P$1 U3.P$49
TXEC-: J3.15(RXCLKINT-) PAD33.P$1 U3.P$50
UART_USB_D+ [USB]: J15.A6(DP1) J15.B6(DP2) PAD49.P$1 U13.P$1(D+)
UART_USB_D- [USB]: J15.A7(DN1) J15.B7(DN2) PAD50.P$1 U13.P$2(D-)
UART_VBUS: D1.A D7.A J15.A4(VBUS) J15.A9(VBUS) J15.B4(VBUS) J15.B9(VBUS) PAD48.P$1
USB_D+ [USB]: PAD45.P$1 R11.2 U1.47(USB_D+)
USB_D- [USB]: PAD46.P$1 R10.2 U1.46(USB_D-)
VCEM-PWM: U3.P$37
VIN [PWR]: C22.2 C23.1 D1.C D4.C R32.2 U26.4(VCC)
VIN2: C52.2 C56.2 L4.1 Q1.3(D) R78.2 U5.6(6-VIN)
VIN+5V [PWR]: C31.2 C32.1 D7.C D8.C D14.C J4.P$1 Q1.2(S) Q5.1(G) Q9.1(G) Q19.2(S) R31.2 R37.2 R38.2 R40.2 R43.2 R49.1 R117.2 U6.1(EN) U6.4(VIN)
XI: C28.1 U3.P$73 X2.1(XIN)
XO: R24.2 U3.P$72
Unconnected: J1.2 J3.1(NC) J3.22(NC) J3.26(NC) J3.30(NC) J5.2 J14.A8(SBU1) J14.B8(SBU2) J15.A8(SBU1) J15.B8(SBU2) P1.P$1 P48.P$1 P49.P$1 SD2.9(CDN) U3.P$39 U3.P$40 U3.P$41 U3.P$42 U3.P$43 U3.P$44 U3.P$45 U3.P$46

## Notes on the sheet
- LCD+TP
- Type-C->USB | RTD2281CL_MCU MIN System
- RP2040_MCU MIN System
- Type-C->URAT0
- Boot:
- Boot=1,正常运行
- RESET=0时，按下Boot-下载模式
- Battery and charging circuit | POWER
- Vout=0.6*(R20/R21 +1)=3.3V
- BAT
- Vout=0.6*(R20/R21 +1)=1.1V
- W25Q32
- W25Q32
- PWR
- 500mA
- Iout=0.2/R29
- LCD-power
- Buzzer | LED Indicator
- TF Card
- Mark
- ADC | I2C | GPIO | PWM | 螺母
- 3.3Vpower，GPIO

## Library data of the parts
B1 = WGH:BEEP_5025
C1-C16 C21 C25 C27-C30 C32 C34-C36 C38-C40 C47-C51 C73 C88 C90-C92 = CrowBot_V1.4:A_XBJ_C0603
C17 C18 C24 C26 C52 C55 C57 C58 C72 = A_xbj:C0603
C19 C20 C22 = CPT_SMD:C0805
C23 C44 = discrete:C*: Ceramic Capacitors
C31 C33 = CrowBot_V1.4:A_XBJ_C0805
C37 = A9G:DISCRETE_C*: Ceramic Capacitors
C41 = A_xbj:DISCRETE_C*: Ceramic Capacitors
C53 C56 = A_xbj:C0805
D1 D2 D4 D6-D8 D14 = diode:DIODE-: DIODE
D3 D15 = Crowtail_SIM1606:DISCRETE_007-LED*
J1 J2 J5 J6 = A_xbj:CONNECTOR_TWIG-4P-2.0-SMD-FEMALE-REINFORCE
J3 = cooper:FPC-0.5-30P-LVDS
J4 = cooper:CON_4PIN_DIP_P2.54
J7 = WGH:2.54-16PIN-WOTIE
J10 = cooper:FPC-6PIN-0.5MM
J14 J15 = WZ3532R024-ESP32-V0.1-20221226:USB_TYPE-C_16PIN
J16 = cooper:PH2.0WT-2PIN
L1 L4 = WZ2432R028-ESP32-V1.2-20231108:L-0530
P1 P48 P49 = crowpi_pow:PAD*
P11-P14 P38 P82 P83 = CrowBot_V1.4:CROWPI_POW_PAD*
PAD1-PAD53 = cooper:PAD
Q1 Q8 Q19 = DFN8:P-MOS-SOT23
Q2 Q3 Q11 = Adafruit_HUZZAH32_ESP32_Feather:SPARKFUN_TRANSISTOR_NPN: Transistor NPN BJT configuration in SOT23 package. MMBT2222 is the common NPN we use. Double check BCE configuration again layout.
Q4 = CrowBot_V1.4:DISCRETE_TRANSISTOR-NPN*: NPN audion
Q5 Q9 = discrete:MOSFET-N: IRLL014: http://www.vishay.com/docs/91319/sihll014.pdf
R1 R2 R5-R7 R9-R11 R14-R24 R27-R31 R35-R41 R43 R45-R47 R53 R81 R82 R85 R98-R101 R108 R109 R116 R117 R121 R122 = Lora_RA-08H_Dev:DISCRETE_R*
R3 R4 R8 R12 R13 R26 R48 R55-R60 R68-R70 R73 R74 R78 R83 R87-R89 R118 = Crowtail-_LED-V2.0-20190615-01:DISCRETE_R*
R32 R66 R84 R96 R97 = A9G:DISCRETE_R*
R44 R50 R51 R80 R86 = cooper:R0603
R49 R79 = discrete:R*
SD2 = Connector:HOLDER-MICROSD-9P
SW2 SW4 = WGH:KEY-6
T1-T4 = DW1000:3M-5
U1 = Lora_RA-08H_Dev:RP2040_RP2040: Raspberry Pi RP2040 MCU 56-pin 32-bit Microcontroller with 264kB of SRAM and external flash support up to 16MB Getting Started with the RP2040 Dual-core ARM Cortex M0+ processor, flexible clock running up to 133 MHz 264kB of SRAM, and QSPI control of common flash memory USB 1.1 Host and Device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; PROD_ID: IC-15502
U2 U4 = Lora_RA-08H_Dev:SELF_W25Q128JV
U3 = cooper:RTD2281CL
U5 = cooper:MT9201
U6 = CrowBot_V1.4:CROWBOT_-V1.0-20220525_A_XBJ_HM3420B
U10 = cooper:BW16
U13 = cooper:CH340N
U26 = DFN8:4054A
X1 X2 = CrowBot_V1.4:A_XBJ_XTAL

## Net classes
0 default: width 0.152 mm, drill 0.305 mm, clearance 0.152 mm
1 PWR: width 0.254 mm
2 GND: width 0.203 mm
3 RS485: width 0.203 mm, clearance 0.203 mm
4 USB: width 0.203 mm, clearance 0.152 mm
5 ANT: width 0.889 mm, clearance 0.203 mm
6 DVI-D0: width 0.203 mm, clearance 0.406 mm to class 0, clearance 0.203 mm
